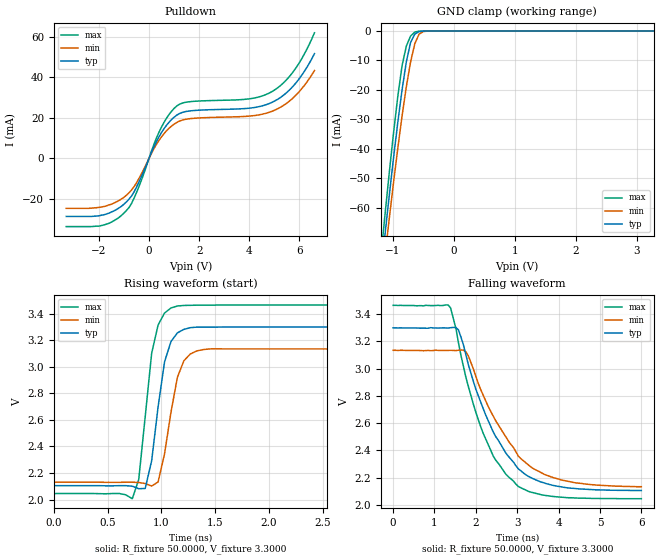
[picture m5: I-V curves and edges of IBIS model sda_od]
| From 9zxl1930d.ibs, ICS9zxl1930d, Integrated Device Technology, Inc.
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|   Model sda_od
[Model]  sda_od
Model_type I/O_open_drain
Polarity   Non-Inverting
Vinl =   0.8000V
Vinh =   2.0000V
Vmeas =  1.6500V
Cref =   0.0F
Rref =   10.0000k
Vref =   3.3000V
C_comp   1.3700pF   1.3700pF   1.3700pF
[Temperature Range]   25.0000   85.0000   -40.0000
[Voltage Range]   3.3000V   3.1350V   3.4650V
[Pullup Reference]   3.3000V   3.1350V   3.4650V
[Pulldown Reference]   0.0V   0.0V   0.0V
[POWER Clamp Reference]   3.3000V   3.1350V   3.4650V
[GND Clamp Reference]   0.0V   0.0V   0.0V
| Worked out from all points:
|   slope of the pulldown table from 0 to 0.495 V, typ, clamps not added: 39 ohm
|   GND clamp passes 1 mA (typ) near -0.64 V on its own axis
|   rising waveform, R_fixture 50.0000, V_fixture 3.3000: 20-80 % time 122ps typ, 130ps min, 120ps max; typ from 2.1 V to 3.3 V
|   falling waveform, R_fixture 50.0000, V_fixture 3.3000: 20-80 % time 1.03ns typ, 1.1ns min, 893ps max; typ from 3.3 V to 2.11 V
[Pulldown]
|Voltage   I(typ)   I(min)   I(max)
-3.3V     -28.6mA    -24.6mA    -33.6mA
-1.8V     -27.8mA    -23.7mA    -32.8mA
-900mV    -21.43mA   -18.13mA   -25.66mA
-500mV    -14.2mA    -12.07mA   -16.88mA
400mV     10.7mA     8.948mA    12.96mA
1.1V      21.3mA     17.71mA    25.8mA
1.7V      23.55mA    19.72mA    28.1mA
4V        24.81mA    20.91mA    29.42mA
4.8V      27.13mA    22.81mA    32.31mA
5.7V      35.01mA    29.35mA    41.94mA
6.2V      43.03mA    36.08mA    51.61mA
6.6V      51.72mA    43.4mA     61.99mA
[GND_clamp]
|Voltage   I(typ)   I(min)   I(max)
-3.3V     -543.2mA   -525.9mA   -564.4mA
-1.2V     -83.07mA   -89.44mA   -77.25mA
-1.13V    -69.33mA   -76.46mA   -62.52mA
-1.06V    -56.02mA   -63.82mA   -48.3mA
-920mV    -31.14mA   -39.94mA   -22.33mA
-850mV    -20.04mA   -28.97mA   -11.85mA
-780mV    -10.54mA   -19.02mA   -5.158mA
-710mV    -3.899mA   -10.54mA   -1.704mA
-640mV    -1.024mA   -4.284mA   -353.9uA
-570mV    -215.4uA   -1.064mA   -49.93uA
-430mV    -5.637uA   -33.74uA   -408.6nA
3.28V     273.7pA    551.6pA    269pA
[Ramp]
| variable   typ   min   max
dV/dt_r  0.7170/0.1217n   0.6024/0.1297n   0.8514/0.1200n
dV/dt_f  0.7164/1.0178n   0.6006/1.1488n   0.8514/0.8927n
R_load = 50.0000
[Rising Waveform]
R_fixture= 50.0000
V_fixture= 3.3000
V_fixture_min= 3.1350
V_fixture_max= 3.4650
|time   V(typ)   V(min)   V(max)
0s        2.105V     2.131V     2.046V
730ps     2.101V     2.131V     2.007V
790ps     2.082V     2.129V     2.152V
850ps     2.084V     2.121V     2.624V
910ps     2.292V     2.102V     3.101V
970ps     2.698V     2.133V     3.314V
1.03ns    3.037V     2.345V     3.404V
1.15ns    3.255V     2.922V     3.457V
1.45ns    3.298V     3.134V     3.463V
6ns       3.3V       3.135V     3.465V
[Falling Waveform]
R_fixture= 50.0000
V_fixture= 3.3000
V_fixture_min= 3.1350
V_fixture_max= 3.4650
|time   V(typ)   V(min)   V(max)
0s        3.3V       3.135V     3.465V
1.39ns    3.301V     3.135V     3.445V
1.58ns    3.284V     3.136V     3.19V
1.76ns    3.101V     3.123V     2.936V
2.18ns    2.705V     2.804V     2.524V
2.48ns    2.502V     2.618V     2.329V
3.03ns    2.264V     2.357V     2.135V
3.39ns    2.192V     2.267V     2.09V
4.06ns    2.133V     2.184V     2.057V
6ns       2.106V     2.134V     2.046V
